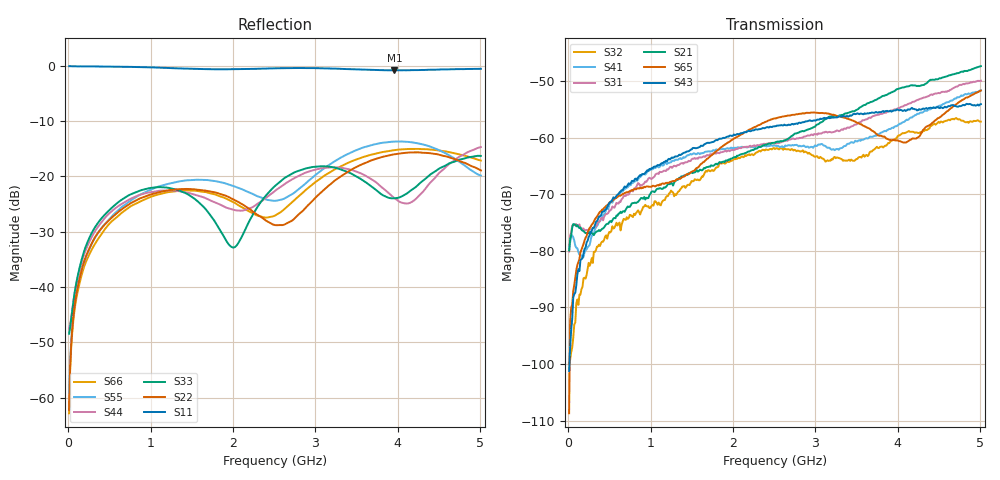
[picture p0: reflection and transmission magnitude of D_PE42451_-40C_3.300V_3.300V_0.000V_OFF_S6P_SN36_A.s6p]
! Device ID: PE42451
! Serial: 36
! Insertion: A
! Temp: -40C
! VDD: 3.300
! Control_Hi: 100.000
! Control_Lo: 0.000
! Logic State: OFF
! Port 1: RFC
! Port 2: RF1
! Port 3: RF2
! Port 4: RF3
! Port 5: RF4
! Port 6: RF5
! V1 = 0.00
! V2 = 3.30
! V3 = 3.30
! V4 = 0.00
! IDD: 1.598340e-05
#  Hz  S  RI  R  50
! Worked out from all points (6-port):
!   401 points, 10 MHz to 5.01 GHz, reference 50 ohm
!   strongest paths, dB at 10 MHz, 1.26 GHz, 2.51 GHz, 3.76 GHz, 5.01 GHz:
!     S43: -101.2, -63.5, -57.9, -55.5, -54.0
!     S65: -108.7, -67.7, -56.5, -59.6, -51.6
!     S21: -79.9, -68.1, -60.9, -53.1, -47.3
!     S31: -80.1, -65.3, -60.8, -55.9, -49.9
!     S41: -80.0, -64.1, -61.4, -59.4, -51.6
!     S32: -99.9, -69.5, -62.0, -61.8, -57.1
!   lowest |S11| = -0.9 dB at 3.96 GHz (marker M1), VSWR 20.26, Z = 2.7 - j15.3 ohm
!   |S11| at or under -10 dB: nowhere
